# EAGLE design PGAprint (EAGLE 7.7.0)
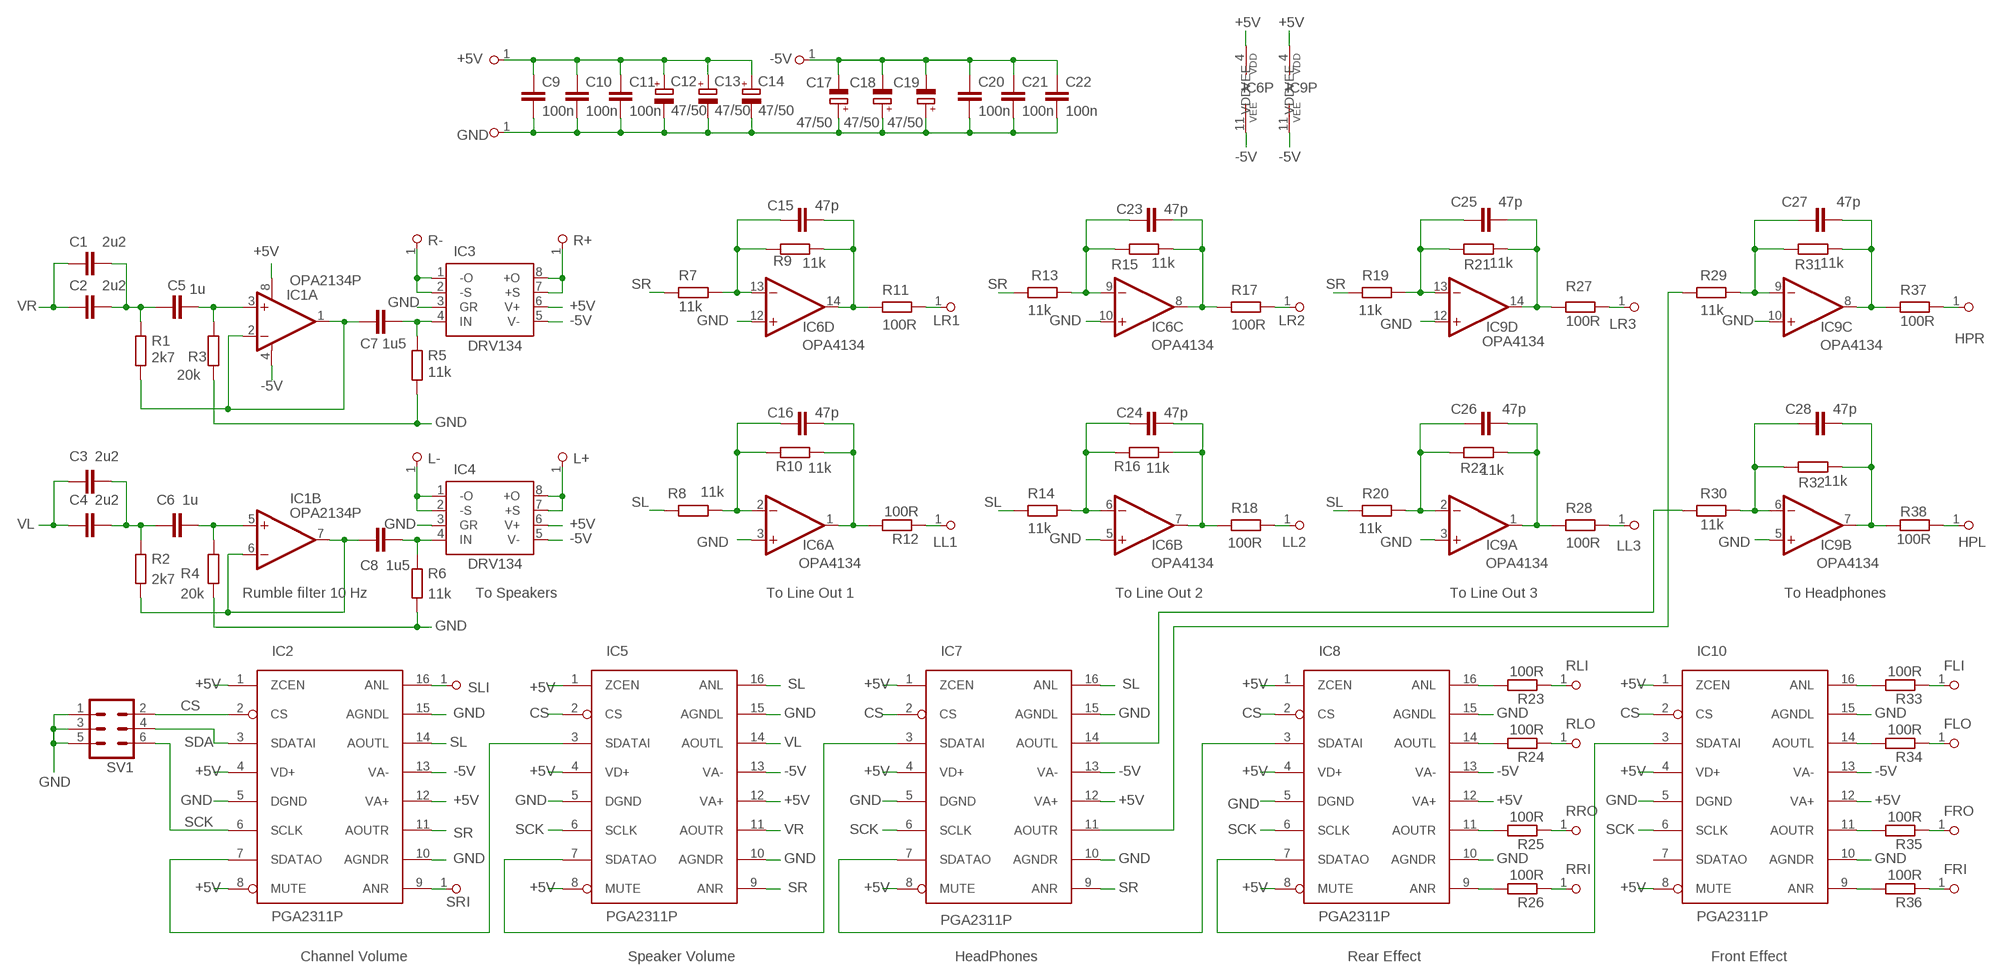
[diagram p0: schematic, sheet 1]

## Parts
+5  PINHDR-1X1  [HDR1X1]
-5  PINHDR-1X1  [HDR1X1]
C1  2u2  C-EU050-075X075  [C050-075X075]
C2  2u2  C-EU050-075X075  [C050-075X075]
C3  2u2  C-EU050-075X075  [C050-075X075]
C4  2u2  C-EU050-075X075  [C050-075X075]
C5  1u  C-EU050-050X075  [C050-050X075]
C6  1u  C-EU050-050X075  [C050-050X075]
C7  1u5  C-EU050-050X075  [C050-050X075]
C8  1u5  C-EU050-050X075  [C050-050X075]
C9  100n  C-EU050-024X044  [C050-024X044]
C10  100n  C-EU050-024X044  [C050-024X044]
C11  100n  C-EU050-024X044  [C050-024X044]
C12  47/50  CPOL-EUE2.5-7  [E2,5-7]
C13  47/50  CPOL-EUE2.5-7  [E2,5-7]
C14  47/50  CPOL-EUE2.5-7  [E2,5-7]
C15  47p  C-EU025-025X050  [C025-025X050]
C16  47p  C-EU025-025X050  [C025-025X050]
C17  47/50  CPOL-EUE2.5-7  [E2,5-7]
C18  47/50  CPOL-EUE2.5-7  [E2,5-7]
C19  47/50  CPOL-EUE2.5-7  [E2,5-7]
C20  100n  C-EU050-024X044  [C050-024X044]
C21  100n  C-EU050-024X044  [C050-024X044]
C22  100n  C-EU050-024X044  [C050-024X044]
C23  47p  C-EU025-025X050  [C025-025X050]
C24  47p  C-EU025-025X050  [C025-025X050]
C25  47p  C-EU025-025X050  [C025-025X050]
C26  47p  C-EU025-025X050  [C025-025X050]
C27  47p  C-EU025-025X050  [C025-025X050]
C28  47p  C-EU025-025X050  [C025-025X050]
FLI  PINHDR-1X1  [HDR1X1]
FLO  PINHDR-1X1  [HDR1X1]
FRI  PINHDR-1X1  [HDR1X1]
FRO  PINHDR-1X1  [HDR1X1]
GND  PINHDR-1X1  [HDR1X1]
HPL  PINHDR-1X1  [HDR1X1]
HPR  PINHDR-1X1  [HDR1X1]
IC1  OPA2134P  [DIL08]
IC2  PGA2311P  [DIL16]
IC3  DRV134  [DIL08]
IC4  DRV134  [DIL08]
IC5  PGA2311P  [DIL16]
IC6  OPA4134  LM124ACN  [DIL14]
IC7  PGA2311P  [DIL16]
IC8  PGA2311P  [DIL16]
IC9  OPA4134  LM124ACN  [DIL14]
IC10  PGA2311P  [DIL16]
L+  PINHDR-1X1  [HDR1X1]
L-  PINHDR-1X1  [HDR1X1]
LL1  PINHDR-1X1  [HDR1X1]
LL2  PINHDR-1X1  [HDR1X1]
LL3  PINHDR-1X1  [HDR1X1]
LR1  PINHDR-1X1  [HDR1X1]
LR2  PINHDR-1X1  [HDR1X1]
LR3  PINHDR-1X1  [HDR1X1]
R1  2k7  R-EU_0204/2V  [0204V]
R2  2k7  R-EU_0204/2V  [0204V]
R3  20k  R-EU_0204/2V  [0204V]
R4  20k  R-EU_0204/2V  [0204V]
R5  11k  R-EU_0204/2V  [0204V]
R6  11k  R-EU_0204/2V  [0204V]
R7  11k  R-EU_0204/2V  [0204V]
R8  11k  R-EU_0204/2V  [0204V]
R9  11k  R-EU_0204/2V  [0204V]
R10  11k  R-EU_0204/2V  [0204V]
R11  100R  R-EU_0204/2V  [0204V]
R12  100R  R-EU_0204/2V  [0204V]
R13  11k  R-EU_0204/2V  [0204V]
R14  11k  R-EU_0204/2V  [0204V]
R15  11k  R-EU_0204/2V  [0204V]
R16  11k  R-EU_0204/2V  [0204V]
R17  100R  R-EU_0204/2V  [0204V]
R18  100R  R-EU_0204/2V  [0204V]
R19  11k  R-EU_0204/2V  [0204V]
R20  11k  R-EU_0204/2V  [0204V]
R21  11k  R-EU_0204/2V  [0204V]
R22  11k  R-EU_0204/2V  [0204V]
R23  100R  R-EU_0204/2V  [0204V]
R24  100R  R-EU_0204/2V  [0204V]
R25  100R  R-EU_0204/2V  [0204V]
R26  100R  R-EU_0204/2V  [0204V]
R27  100R  R-EU_0204/2V  [0204V]
R28  100R  R-EU_0204/2V  [0204V]
R29  11k  R-EU_0204/2V  [0204V]
R30  11k  R-EU_0204/2V  [0204V]
R31  11k  R-EU_0204/2V  [0204V]
R32  11k  R-EU_0204/2V  [0204V]
R33  100R  R-EU_0204/2V  [0204V]
R34  100R  R-EU_0204/2V  [0204V]
R35  100R  R-EU_0204/2V  [0204V]
R36  100R  R-EU_0204/2V  [0204V]
R37  100R  R-EU_0204/2V  [0204V]
R38  100R  R-EU_0204/2V  [0204V]
R+  PINHDR-1X1  [HDR1X1]
R-  PINHDR-1X1  [HDR1X1]
RLI  PINHDR-1X1  [HDR1X1]
RLO  PINHDR-1X1  [HDR1X1]
RRI  PINHDR-1X1  [HDR1X1]
RRO  PINHDR-1X1  [HDR1X1]
SL  PINHDR-1X1  [HDR1X1]
SR  PINHDR-1X1  [HDR1X1]
SV1  PINHD-3X2  [MA03-2]

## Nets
+5V: +5.1 C9.1 C10.1 C11.1 C12.+ C13.+ C14.+ IC1.8(A:V+) IC2.1(ZCEN) IC2.4(VD+) IC2.8(MUTE) IC2.12(VA+) IC3.6(V+) IC4.6(V+) IC5.1(ZCEN) IC5.4(VD+) IC5.8(MUTE) IC5.12(VA+) IC6.4(P:VDD) IC7.1(ZCEN) IC7.4(VD+) IC7.8(MUTE) IC7.12(VA+) IC8.1(ZCEN) IC8.4(VD+) IC8.8(MUTE) IC8.12(VA+) IC9.4(P:VDD) IC10.1(ZCEN) IC10.4(VD+) IC10.8(MUTE) IC10.12(VA+)
-5V: -5.1 C17.- C18.- C19.- C20.1 C21.1 C22.1 IC1.4(A:V-) IC2.13(VA-) IC3.5(V-) IC4.5(V-) IC5.13(VA-) IC6.11(P:VEE) IC7.13(VA-) IC8.13(VA-) IC9.11(P:VEE) IC10.13(VA-)
CS: IC2.2(CS) IC5.2(CS) IC7.2(CS) IC8.2(CS) IC10.2(CS) SV1.2
FLI: FLI.1 R33.1
FLO: FLO.1 R34.1
FRI: FRI.1 R36.1
FRO: FRO.1 R35.1
GND: C9.2 C10.2 C11.2 C12.- C13.- C14.- C17.+ C18.+ C19.+ C20.2 C21.2 C22.2 GND.1 IC2.5(DGND) IC2.10(AGNDR) IC2.15(AGNDL) IC3.3(GR) IC4.3(GR) IC5.5(DGND) IC5.10(AGNDR) IC5.15(AGNDL) IC6.3(A:+IN) IC6.5(B:+IN) IC6.10(C:+IN) IC6.12(D:+IN) IC7.5(DGND) IC7.10(AGNDR) IC7.15(AGNDL) IC8.5(DGND) IC8.10(AGNDR) IC8.15(AGNDL) IC9.3(A:+IN) IC9.5(B:+IN) IC9.10(C:+IN) IC9.12(D:+IN) IC10.5(DGND) IC10.10(AGNDR) IC10.15(AGNDL) R3.1 R4.2 R5.2 R6.2 SV1.1 SV1.3 SV1.5
HPL: HPL.1 R38.1
HPR: HPR.1 R37.1
L+: IC4.7(+S) IC4.8(+O) L+.1
L-: IC4.1(-O) IC4.2(-S) L-.1
LL1: LL1.1 R12.1
LL2: LL2.1 R18.1
LL3: LL3.1 R28.1
LR1: LR1.1 R11.1
LR2: LR2.1 R17.1
LR3: LR3.1 R27.1
N$1: C3.2 C4.2 C6.1 R2.1
N$3: C1.2 C2.2 C5.1 R1.1
N$4: C5.2 IC1.3(A:+IN) R3.2
N$5: C6.2 IC1.5(B:+IN) R4.1
N$6: C8.1 IC1.6(B:-IN) IC1.7(B:OUT) R2.2
N$7: IC2.7(SDATAO) IC5.3(SDATAI)
N$9: IC8.16(ANL) R23.2
N$11: C8.2 IC4.4(IN) R6.1
N$14: C7.2 IC3.4(IN) R5.1
N$15: C7.1 IC1.1(A:OUT) IC1.2(A:-IN) R1.2
N$17: IC8.14(AOUTL) R24.2
N$20: IC8.11(AOUTR) R25.2
N$23: C16.1 IC6.2(A:-IN) R8.1 R10.2
N$24: IC5.7(SDATAO) IC7.3(SDATAI)
N$25: IC8.9(ANR) R26.2
N$26: C16.2 IC6.1(A:OUT) R10.1 R12.2
N$29: C15.2 IC6.14(D:OUT) R9.1 R11.2
N$32: IC10.16(ANL) R33.2
N$34: C15.1 IC6.13(D:-IN) R7.1 R9.2
N$35: C28.1 IC9.6(B:-IN) R30.1 R32.2
N$36: IC10.14(AOUTL) R34.2
N$37: IC10.11(AOUTR) R35.2
N$38: IC10.9(ANR) R36.2
N$40: IC7.7(SDATAO) IC8.3(SDATAI)
N$44: IC7.14(AOUTL) R30.2
N$45: C24.1 IC6.6(B:-IN) R14.1 R16.2
N$46: C23.1 IC6.9(C:-IN) R13.1 R15.2
N$47: IC7.11(AOUTR) R29.2
N$49: C27.1 IC9.9(C:-IN) R29.1 R31.2
N$50: C23.2 IC6.8(C:OUT) R15.1 R17.2
N$51: C24.2 IC6.7(B:OUT) R16.1 R18.2
N$56: C26.1 IC9.2(A:-IN) R20.1 R22.2
N$61: C25.1 IC9.13(D:-IN) R19.1 R21.2
N$64: C26.2 IC9.1(A:OUT) R22.1 R28.2
N$66: C28.2 IC9.7(B:OUT) R32.1 R38.2
N$67: C25.2 IC9.14(D:OUT) R21.1 R27.2
N$68: IC8.7(SDATAO) IC10.3(SDATAI)
N$73: C27.2 IC9.8(C:OUT) R31.1 R37.2
R+: IC3.7(+S) IC3.8(+O) R+.1
R-: IC3.1(-O) IC3.2(-S) R-.1
RLI: R23.1 RLI.1
RLO: R24.1 RLO.1
RRI: R26.1 RRI.1
RRO: R25.1 RRO.1
SCK: IC2.6(SCLK) IC5.6(SCLK) IC7.6(SCLK) IC8.6(SCLK) IC10.6(SCLK) SV1.6
SDA: IC2.3(SDATAI) SV1.4
SL: IC2.14(AOUTL) IC5.16(ANL) IC7.16(ANL) R8.2 R14.2 R20.2
SLI: IC2.16(ANL) SL.1
SR: IC2.11(AOUTR) IC5.9(ANR) IC7.9(ANR) R7.2 R13.2 R19.2
SRI: IC2.9(ANR) SR.1
VL: C3.1 C4.1 IC5.14(AOUTL)
VR: C1.1 C2.1 IC5.11(AOUTR)
Unconnected: IC10.7(SDATAO)

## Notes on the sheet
- Rumble filter 10 Hz | To Speakers | To Line Out 1 | To Line Out 2 | To Line Out 3 | To Headphones
- Channel Volume | Speaker Volume | HeadPhones | Rear Effect | Front Effect

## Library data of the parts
+5 -5 FLI FLO FRI FRO GND HPL HPR L+ L- LL1-LL3 LR1-LR3 R+ R- RLI RLO RRI RRO SL SR = Connector:PINHDR-1X1
C1-C11 C15 C16 C20-C28 = Passive:C-EU: CAPACITOR, European symbol
C12-C14 C17-C19 = Passive:CPOL-EU: POLARIZED CAPACITOR, European symbol
IC1 = IC_Lin:OPA2134: Operational Amplifier
IC2 IC5 IC7 IC8 IC10 = IC_MixMode:PGA2311: Stereo Volume Control
IC3 IC4 = IC_Lin:DRV134
IC6 IC9 = IC_Lin:LM124: Quad Op Amp
R1-R38 = AJANLIB:R-EU_: RESISTOR, European symbol
SV1 = Header:PINHD-3X2: PIN HEADER

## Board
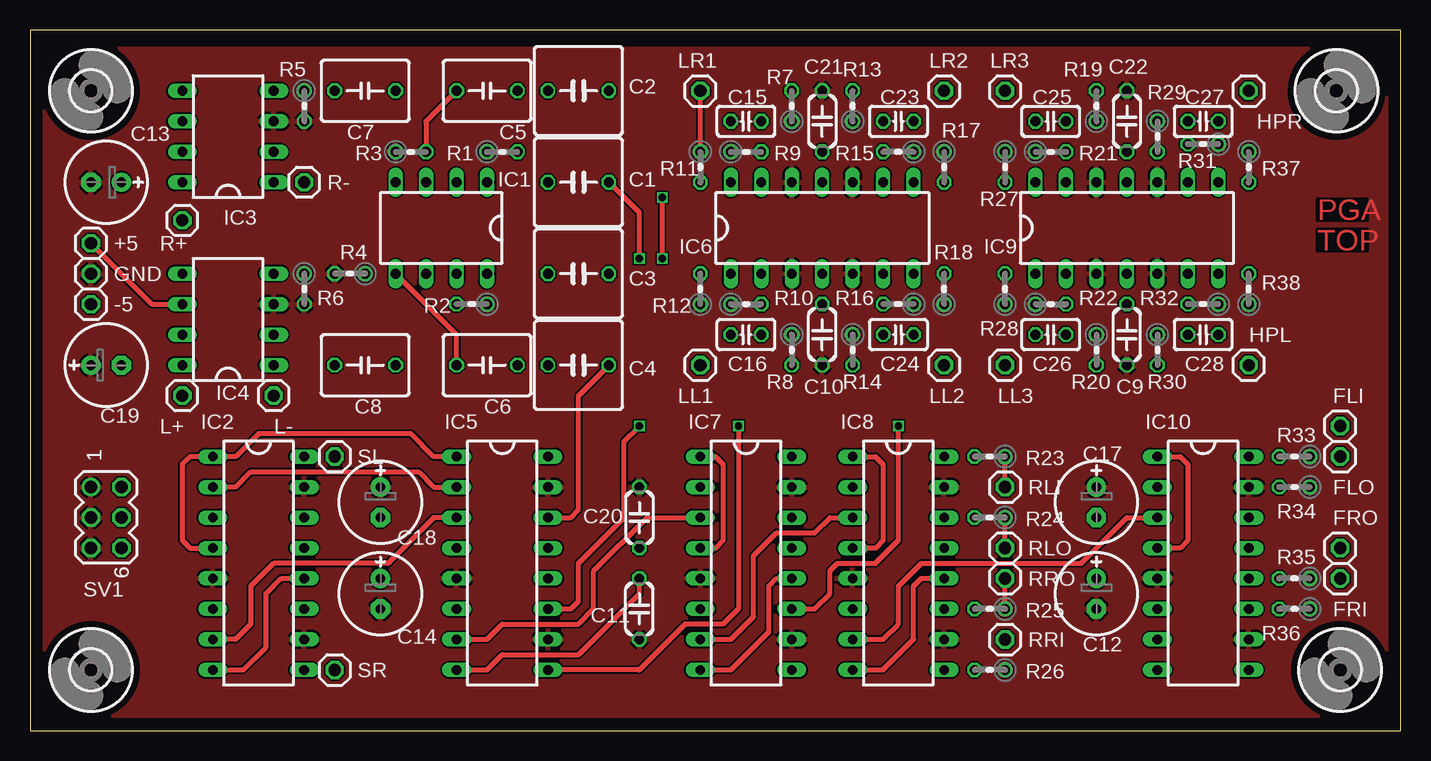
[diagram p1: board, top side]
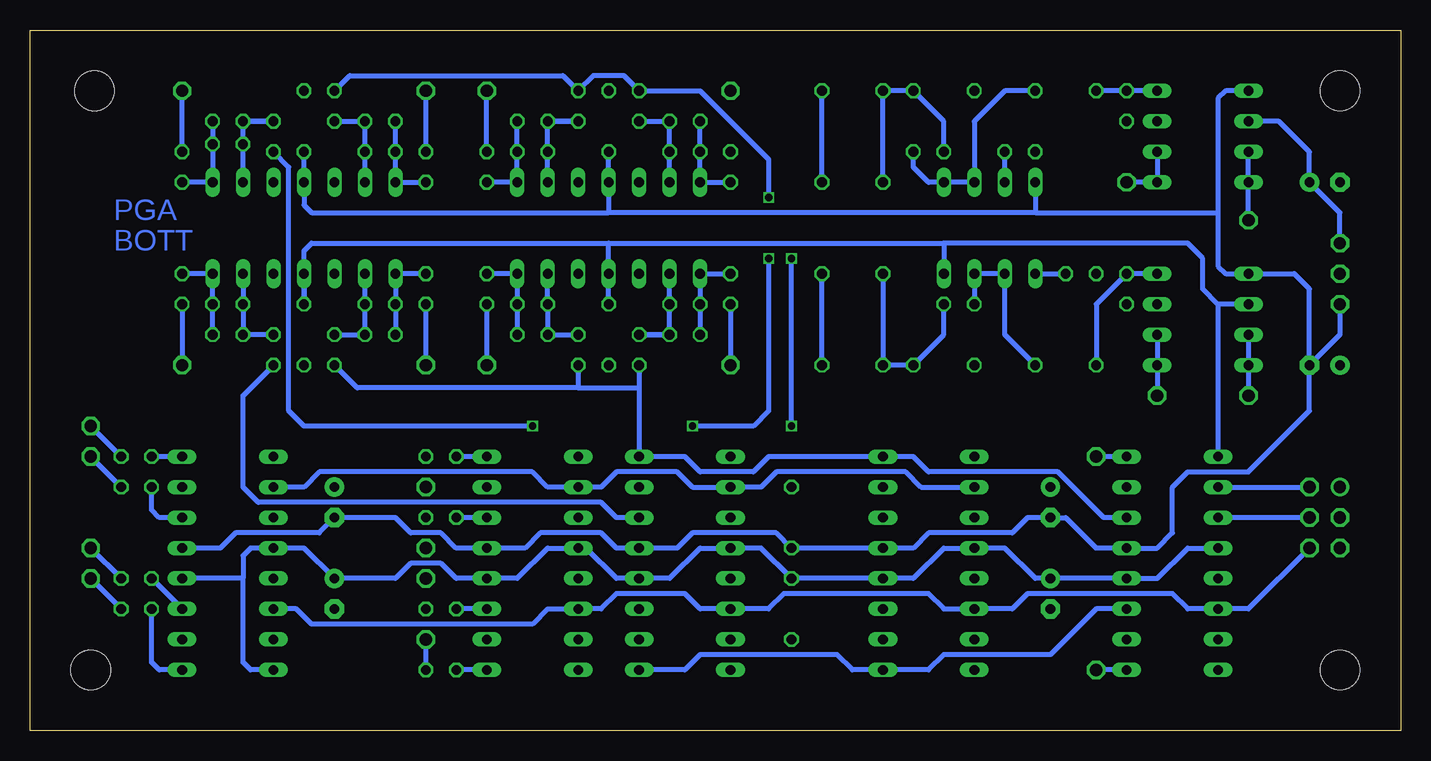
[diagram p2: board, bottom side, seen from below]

Size 114.28 x 58.41 mm. Coordinates in mm from the lower left corner, seen from the top.
Outline: 0,0 114.28,0 114.28,58.41 0,58.41 0,0
Copper layers (1*16): Top 0.018mm / dielectric 1.55mm / Bottom 0.018mm
Design rules "eC_2Layer_PClass6_BaseCopperO18_eCDefault": minimum track width 0.15mm, minimum drill 0.35mm, track to track 0.15mm, track to pad 0.15mm, pad to pad 0.15mm, via to via 0.15mm, smd to smd 0mil, copper to edge 0.25mm, drill to drill 0.35mm, minimum pad ring 0.175mm, minimum via ring 0.125mm, stop-mask expansion 0mil, vias tented up to drill 0.45mm, thermal gap 0.2mm

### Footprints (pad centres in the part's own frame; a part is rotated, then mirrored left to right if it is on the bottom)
HDR1X1 = drill 1.016 octagon: 1 0,0
C050-075X075 = drill 0.813 octagon: 1 -2.54,0; 2 2.54,0
C050-050X075 = drill 0.813 octagon: 1 -2.54,0; 2 2.54,0
C050-024X044 = drill 0.813 octagon: 1 -2.54,0; 2 2.54,0
E2,5-7 = drill 0.813 pad 1.6: + -1.27,0 | drill 0.813 pad 1.6 octagon: - 1.27,0
C025-025X050 = drill 0.813 octagon: 1 -1.27,0; 2 1.27,0
DIL08 = drill 0.813 long: 1 -3.81,-3.81; 2 -1.27,-3.81; 3 1.27,-3.81; 4 3.81,-3.81; 5 3.81,3.81; 6 1.27,3.81; 7 -1.27,3.81; 8 -3.81,3.81
DIL16 = drill 0.813 long: 1 -8.89,-3.81; 2 -6.35,-3.81; 3 -3.81,-3.81; 4 -1.27,-3.81; 5 1.27,-3.81; 6 3.81,-3.81; 7 6.35,-3.81; 8 8.89,-3.81; 9 8.89,3.81; 10 6.35,3.81; 11 3.81,3.81; 12 1.27,3.81; 13 -1.27,3.81; 14 -3.81,3.81; 15 -6.35,3.81; 16 -8.89,3.81
DIL14 = drill 0.813 long: 1 -7.62,-3.81; 2 -5.08,-3.81; 3 -2.54,-3.81; 4 0,-3.81; 5 2.54,-3.81; 6 5.08,-3.81; 7 7.62,-3.81; 8 7.62,3.81; 9 5.08,3.81; 10 2.54,3.81; 11 0,3.81; 12 -2.54,3.81; 13 -5.08,3.81; 14 -7.62,3.81
0204V = drill 0.813 octagon: 1 -1.27,0; 2 1.27,0
MA03-2 = drill 1.016: 1 -2.54,-1.27 | drill 1.016 octagon: 2 -2.54,1.27; 3 0,-1.27; 4 0,1.27; 5 2.54,-1.27; 6 2.54,1.27
3,3 = hole 3.3: 0,0

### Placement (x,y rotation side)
+5  5.08,40.64 0 top
-5  5.08,35.56 0 top
C1  45.72,45.72 180 top
C2  45.72,53.34 180 top
C3  45.72,38.1 180 top
C4  45.72,30.48 180 top
C5  38.1,53.34 180 top
C6  38.1,30.48 180 top
C7  27.94,53.34 180 top
C8  27.94,30.48 180 top
C9  91.44,33.02 270 top
C10  66.04,33.02 270 top
C11  50.8,10.16 270 top
C12  88.9,11.43 270 top
C13  6.35,45.72 180 top
C14  29.21,11.43 270 top
C15  59.69,50.8 180 top
C16  59.69,33.02 180 top
C17  88.9,19.05 270 top
C18  29.21,19.05 270 top
C19  6.35,30.48 0 top
C20  50.8,17.78 90 top
C21  66.04,50.8 90 top
C22  91.44,50.8 90 top
C23  72.39,50.8 0 top
C24  72.39,33.02 0 top
C25  85.09,50.8 180 top
C26  85.09,33.02 180 top
C27  97.79,50.8 0 top
C28  97.79,33.02 0 top
FLI  109.22,25.4 0 top
FLO  109.22,22.86 0 top
FRI  109.22,12.7 0 top
FRO  109.22,15.24 0 top
GND  5.08,38.1 0 top
HPL  101.6,30.48 0 top
HPR  101.6,53.34 0 top
IC1  34.29,41.91 180 top
IC2  19.05,13.97 270 top
IC3  16.51,49.53 90 top
IC4  16.51,34.29 90 top
IC5  39.37,13.97 270 top
IC6  66.04,41.91 0 top
IC7  59.69,13.97 270 top
IC8  72.39,13.97 270 top
IC9  91.44,41.91 0 top
IC10  97.79,13.97 270 top
L+  12.7,27.94 90 top
L-  20.32,27.94 90 top
LL1  55.88,30.48 0 top
LL2  76.2,30.48 0 top
LL3  81.28,30.48 0 top
LR1  55.88,53.34 0 top
LR2  76.2,53.34 0 top
LR3  81.28,53.34 0 top
R1  39.37,48.26 0 top
R2  36.83,35.56 180 top
R3  31.75,48.26 0 top
R4  26.67,38.1 180 top
R5  22.86,52.07 270 top
R6  22.86,36.83 270 top
R7  63.5,52.07 90 top
R8  63.5,31.75 270 top
R9  59.69,48.26 0 top
R10  59.69,35.56 0 top
R11  55.88,46.99 270 top
R12  55.88,36.83 90 top
R13  68.58,52.07 90 top
R14  68.58,31.75 270 top
R15  72.39,48.26 180 top
R16  72.39,35.56 180 top
R17  76.2,46.99 270 top
R18  76.2,36.83 90 top
R19  88.9,52.07 90 top
R20  88.9,31.75 270 top
R21  85.09,48.26 0 top
R22  85.09,35.56 0 top
R23  80.01,22.86 180 top
R24  80.01,17.78 180 top
R25  80.01,10.16 180 top
R26  80.01,5.08 180 top
R27  81.28,46.99 270 top
R28  81.28,36.83 90 top
R29  93.98,49.53 270 top
R30  93.98,31.75 270 top
R31  97.79,48.9 180 top
R32  97.79,35.56 180 top
R33  105.41,22.86 180 top
R34  105.41,20.32 180 top
R35  105.41,12.7 180 top
R36  105.41,10.16 180 top
R37  101.6,46.99 270 top
R38  101.6,36.83 90 top
R+  12.7,42.55 90 top
R-  22.86,45.72 90 top
RLI  81.28,20.32 0 top
RLO  81.28,15.24 0 top
RRI  81.28,7.62 0 top
RRO  81.28,12.7 0 top
SL  25.4,22.86 0 top
SR  25.4,5.08 0 top
SV1  6.35,17.78 270 top
U$3  [3,3]  5.08,5.08 0 top
U$4  [3,3]  109.22,5.08 0 top
U$5  [3,3]  5.08,53.34 0 top
U$6  [3,3]  108.9,53.34 0 top

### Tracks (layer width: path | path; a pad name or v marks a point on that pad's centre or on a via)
+5V
  Top 0.406: IC8.8 71.12,5.08 73.66,7.62 73.66,12.06 74.3,12.7 IC8.12 | IC7.8 58.42,5.08 61.59,8.26 61.59,12.06 62.23,12.7 IC7.12 | IC2.8 17.78,5.08 19.68,6.99 19.68,11.43 20.95,12.7 IC2.12 | IC5.8 38.1,5.08 39.37,6.35 45.72,6.35 50.8,11.43 C11.1 | IC2.4 13.34,15.24 12.7,15.88 12.7,22.23 13.34,22.86 IC2.1 17.14,22.86 19.05,24.77 31.75,24.77 33.66,22.86 IC5.1 | IC7.1 57.15,22.86 57.78,22.23 57.78,15.88 57.15,15.24 IC7.4 | IC8.1 70.48,22.86 71.12,22.23 71.12,15.88 70.48,15.24 IC8.4 | IC10.1 95.89,22.86 96.52,22.23 96.52,15.88 95.89,15.24 IC10.4 | +5.1 10.16,35.56 IC4.6
  Bottom 0.406: IC2.4 17.78,15.24 20.32,12.7 IC2.12 C14.+ 30.48,12.7 33.02,15.24 IC5.4 38.1,15.24 40.64,12.7 IC5.12 C11.1 53.34,15.24 IC7.4 58.42,15.24 60.96,12.7 IC7.12 65.41,12.7 67.94,15.24 IC8.4 71.12,15.24 73.66,12.7 IC8.12 78.74,12.7 80.01,13.97 82.55,13.97 83.82,12.7 C12.+ 91.44,15.24 IC10.4 95.89,15.24 96.52,14.61 96.52,12.7 | IC10.8 95.89,5.08 96.52,5.71 96.52,12.7 | 96.52,12.7 IC10.12 | IC6.4 C10.1 66.04,40.64 | 66.04,40.64 38.1,40.64 | IC9.4 C9.1 91.44,40.01 90.81,40.64 66.04,40.64 | 38.1,40.64 IC1.8 | 15.24,35.56 16.51,36.83 16.51,39.37 17.78,40.64 38.1,40.64 | 15.24,35.56 IC2.1 | +5.1 5.08,43.18 C13.+ 7.62,48.26 10.16,50.8 IC3.6 | IC4.6 15.24,35.56
-5V
  Bottom 0.406: IC10.13 98.42,15.24 97.16,16.51 90.17,16.51 C17.- 83.82,17.78 82.55,16.51 80.01,16.51 78.74,15.24 IC8.13 73.03,15.24 71.75,16.51 66.67,16.51 65.41,15.24 IC7.13 60.33,15.24 59.05,16.51 52.07,16.51 C20.1 IC5.13 40.64,15.24 39.37,16.51 32.38,16.51 31.11,17.78 C18.- 27.94,17.78 25.4,15.24 IC2.13 20.32,15.24 19.05,16.51 19.05,20.32 17.78,21.59 12.7,21.59 7.62,26.67 C19.- | C21.1 IC6.11 66.04,43.18 | 66.04,43.18 90.81,43.18 91.44,43.81 IC9.11 C22.1 | IC1.4 30.48,43.18 | 30.48,43.18 66.04,43.18 | 30.48,43.18 15.24,43.18 | 15.24,43.18 15.24,38.73 14.61,38.1 IC4.5 8.89,38.1 7.62,36.83 C19.- | 15.24,43.18 15.24,52.7 14.61,53.34 IC3.5 | C19.- 5.08,33.02 -5.1
CS
  Top 0.406: IC5.2 33.66,20.32 32.38,21.59 18.41,21.59 17.14,20.32 IC2.2
  Bottom 0.406: IC10.2 91.44,20.32 90.17,21.59 72.39,21.59 71.12,20.32 IC8.2 66.67,20.32 65.41,21.59 60.33,21.59 59.05,20.32 IC7.2 53.34,20.32 52.07,21.59 41.27,21.59 40.01,20.32 IC5.2 | IC2.2 SV1.2
FLI
  Bottom 0.406: R33.1 FLI.1
FLO
  Bottom 0.406: R34.1 FLO.1
FRI
  Bottom 0.406: R36.1 FRI.1
FRO
  Bottom 0.406: FRO.1 R35.1
GND
  pour Top: 1.27,56.83 113.03,56.83 113.03,1.27 1.27,1.27
HPL
  Bottom 0.406: R38.1 HPL.1
HPR
  Bottom 0.406: R37.1 HPR.1
L+
  Bottom 0.406: IC4.7 IC4.8 L+.1
L-
  Bottom 0.406: IC4.2 IC4.1 L-.1
LL1
  Bottom 0.406: R12.1 LL1.1
LL2
  Bottom 0.406: R18.1 LL2.1
LL3
  Bottom 0.406: LL3.1 R28.1
LR1
  Top 0.406: R11.1 LR1.1
LR2
  Bottom 0.406: R17.1 LR2.1
LR3
  Bottom 0.406: R27.1 LR3.1
N$1
  Bottom 0.406: R2.1 38.1,33.02 C6.1 C4.2 C3.2
N$3
  Bottom 0.406: R1.1 38.1,50.8 C5.1 C2.2 C1.2
N$4
  Top 0.406: C5.2 33.02,50.8 R3.2
  Bottom 0.406: IC1.3 R3.2
N$5
  Top 0.406: C6.2 35.56,33.02 IC1.5
  Bottom 0.406: IC1.5 R4.1
N$6
  Bottom 0.406: C8.1 33.02,33.02 IC1.6 IC1.7 R2.2
N$7
  Top 0.406: IC5.3 33.66,17.78 29.84,13.97 20.32,13.97 18.41,12.06 18.41,8.89 17.14,7.62 IC2.7
N$9
  Bottom 0.406: IC8.16 R23.2
N$11
  Bottom 0.406: C8.2 25.4,35.56 R6.1 IC4.4
N$14
  Bottom 0.406: C7.2 R5.1 IC3.4
N$15
  Bottom 0.406: C7.1 33.02,53.34 35.56,50.8 IC1.2 IC1.1 39.37,45.72 40.64,46.99 R1.2
N$17
  Bottom 0.406: IC8.14 R24.2
N$20
  Bottom 0.406: IC8.11 R25.2
N$23
  Bottom 0.406: C16.1 R8.1 C16.1 | C16.1 61.59,33.02 C16.1 | C16.1 R10.2 IC6.2
N$24
  Top 0.406: IC5.7 38.1,7.62 39.37,8.89 45.72,8.89 46.99,10.16 46.99,13.34 51.44,17.78 IC7.3
N$25
  Bottom 0.406: IC8.9 R26.2
N$26
  Bottom 0.406: R12.2 IC6.1 R10.1 C16.2
N$29
  Bottom 0.406: R11.2 IC6.14 R9.1 C15.2
N$32
  Bottom 0.406: IC10.16 R33.2
N$34
  Bottom 0.406: IC6.13 R9.2 C15.1 R7.1
N$35
  Bottom 0.406: IC9.6 R32.2 C28.1 R30.1
N$36
  Bottom 0.406: IC10.14 103.5,17.78 104.14,18.41 R34.2
N$37
  Bottom 0.406: R35.2 IC10.11
N$38
  Bottom 0.406: IC10.9 103.5,5.08 104.14,5.71 R36.2
N$40
  Top 0.406: IC7.7 58.42,7.62 60.33,9.53 60.33,14.61 62.23,16.51 65.41,16.51 66.67,17.78 IC8.3
N$44
  Bottom 0.406: IC7.14 65.41,17.78 66.67,19.05 95.25,19.05 96.52,20.32 96.52,27.94 R30.2
N$45
  Bottom 0.406: C24.1 R14.1 C24.1 | IC6.6 R16.2 C24.1
N$46
  Bottom 0.406: IC6.9 R15.2 C23.1 | C23.1 R13.1 C23.1
N$47  (via drill 0.6)
  Top 0.406: IC7.11 65.41,10.16 66.67,11.43 66.67,13.34 67.31,13.97 70.48,13.97 72.39,15.88 v72.39,25.4
  Bottom 0.406: v72.39,25.4 91.44,25.4 92.71,26.67 92.71,46.99 R29.2
N$49
  Bottom 0.406: IC9.9 R31.2 C27.1 | C27.1 R29.1 C27.1
N$50
  Bottom 0.406: C23.2 R15.1 IC6.8 R17.2
N$51
  Bottom 0.406: C24.2 R16.1 IC6.7 R18.2
N$56
  Bottom 0.406: R20.1 C26.1 R22.2 IC9.2
N$61
  Bottom 0.406: IC9.13 R21.2 C25.1 R19.1
N$64
  Bottom 0.406: R28.2 IC9.1 R22.1 C26.2
N$66
  Bottom 0.406: C28.2 R32.1 IC9.7 R38.2
N$67
  Bottom 0.406: R27.2 IC9.14 R21.1 C25.2
N$68
  Top 0.406: IC8.7 71.12,7.62 72.39,8.89 72.39,12.06 74.3,13.97 87.63,13.97 91.44,17.78 IC10.3
N$73
  Bottom 0.406: C27.2 R31.1 IC9.8 R37.2
R+
  Bottom 0.406: R+.1 IC3.8 IC3.7
R-
  Bottom 0.406: IC3.2 IC3.1 R-.1
RLI
  Top 0.406: RLI.1 R23.1
RLO
  Top 0.406: RLO.1 R24.1
RRI
  Bottom 0.406: R26.1 RRI.1
RRO
  Top 0.406: R25.1 RRO.1
SCK
  Bottom 0.406: SV1.6 12.7,10.16 IC2.6 17.78,10.16 19.05,11.43 31.11,11.43 32.38,10.16 IC5.6 38.1,10.16 39.37,11.43 51.44,11.43 52.7,10.16 IC7.6 58.42,10.16 59.69,11.43 65.41,11.43 66.67,10.16 IC8.6 71.12,10.16 72.39,8.89 90.81,8.89 92.08,10.16 IC10.6
SDA
  Bottom 0.406: SV1.4 IC2.3
SL
  Bottom 0.406: IC2.14 24.77,17.78 28.57,21.59 39.37,21.59 40.64,22.86 IC5.16 52.7,22.86 53.98,21.59 58.42,21.59 59.69,22.86 IC7.16 63.5,28.57 | 68.58,28.57 63.5,28.57 | R8.2 63.5,28.57 | R14.2 68.58,28.57 | 68.58,28.57 87,28.57 R20.2
SLI
  Bottom 0.406: IC2.16 SL.1
SR  (via drill 0.6)
  Top 0.406: v52.7,44.45 v52.7,39.37 | v59.05,25.4 59.05,10.16 57.78,8.89 54.61,8.89 50.8,5.08 IC5.9
  Bottom 0.406: IC2.11 25.4,10.16 29.21,6.35 38.1,6.35 39.37,5.08 IC5.9 45.72,5.08 46.99,6.35 58.42,6.35 59.69,5.08 IC7.9 | R19.2 87.63,54.61 69.85,54.61 R13.2 67.31,54.61 64.77,54.61 R7.2 58.42,53.34 52.7,47.62 v52.7,44.45 | v52.7,39.37 52.7,26.67 53.98,25.4 v59.05,25.4
SRI
  Bottom 0.406: IC2.9 SR.1
VL
  Top 0.406: IC5.14 45.09,17.78 45.72,18.41 45.72,27.94 C4.1
  Bottom 0.406: C4.1 C3.1
VR  (via drill 0.6)
  Top 0.406: IC5.11 45.09,10.16 45.72,10.79 45.72,13.97 49.53,17.78 49.53,24.13 v50.8,25.4 | v50.8,39.37 50.8,43.18 C1.1
  Bottom 0.406: v50.8,25.4 v50.8,39.37 | C1.1 C2.1

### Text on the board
Top: PGA | TOP
Bottom: PGA | BOTT
tNames: 1 | 6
